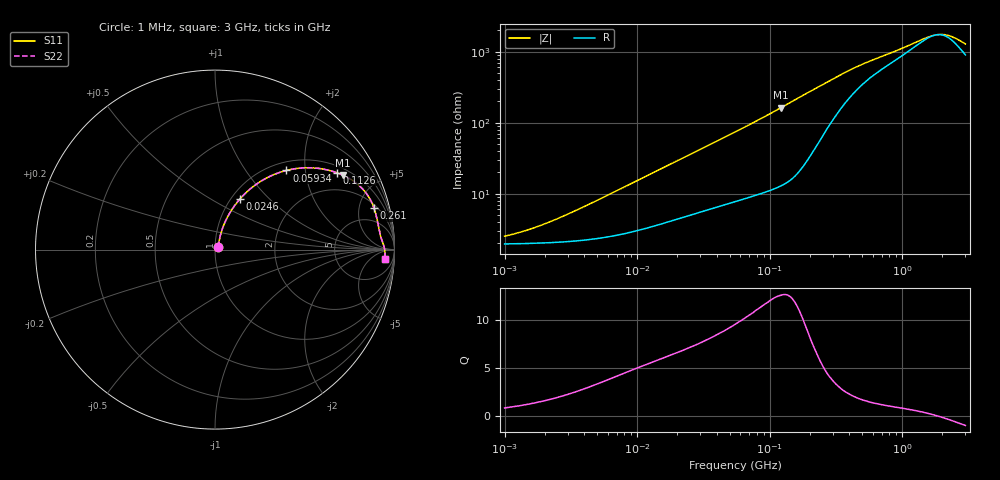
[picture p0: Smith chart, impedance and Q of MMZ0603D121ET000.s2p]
! S-Parameter Data Generated by TDK Corporation
! Copyright(C) 2025 TDK Corporation.
! All Rights Reserved.
! TDK P/N: MMZ0603D121ET000 (Chip Bead)
! Property: |Z|=120ohm at 100MHz
! Size(LxWxT): 0.6x0.3x0.3mm
! Model Type: s2p (Touchstone File Format Version 1.0)
! Frequency: DC=Yes Start=1MHz Stop=3000MHz 202points Log-sweep
! Model Generated on Feb. 6, 2025
! Terms and conditions regarding TDK Simulation Models:
! 1)This simulation model is being provided solely for informational
!  purposes. Please refer to the specifications of the products in
!  terms of detailed characteristics of such products.
! 2)In no event shall TDK Corporation of any of its subsidiaries be
!  liable for any loss or damage arising, directly or indirectly,
!  from any information contained in this simulation model, including,
!  but not limited to loss or damages arising from any inaccuracies,
!  omissions or errors in connection with such information.
! 3)Any and all copyrights on this simulation model are owned by
!  TDK Corporation.  Duplication or redistribution of this simulation
!  model without prior written permission from TDK Corporation
!  is prohibited.
! 4)This simulation model is subject to any modification or change
!  without any prior notice.
! 5)Neither TDK Corporation nor any of its subsidiaries shall make any
!  warranty, express or implied, including but not limited to the
!  correctness, implied warranties of merchantability and fitness for
!  a particular purpose with respect to this simulation models.
! 6)The use of this simulation model shall be deemed to have consented
!  to the terms and conditions hereof.
! Port Assignments:
!  1 ---@@@--- 2
! Applicable Conditions:
!  Temperature = 25 degC
!  DC Bias Current = 0 A
!  Small Signal Operation
# Hz S MA R 50
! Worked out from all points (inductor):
!   201 points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, 1 MHz to 3 GHz, reference 50 ohm
!   read as one part in series: L = 245 nH near 4.398 MHz
!   highest Q = 12.6 at 122 MHz (marker M1), where L = 211 nH
!   self-resonance near 1.818 GHz
!   S11 on the Smith chart (normalised r, x): 1 MHz: 1.04, +0.03; 24.6 MHz: 1.10, +0.69; 59.34 MHz: 1.16, +1.58; 112.6 MHz: 1.24, +2.98; 261 MHz: 2.46, +6.99; 3 GHz: 19, -18
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1000000  0.02469 37.9  0.9806 -0.9  0.9806 -0.9  0.02469 37.9
1377479  0.02886 46.5  0.9803 -1.2  0.9803 -1.2  0.02886 46.5
1897447  0.03537 54.3  0.9798 -1.7  0.9798 -1.7  0.03537 54.3
3900413  0.06306 66.6  0.9767 -3.4  0.9767 -3.4  0.06306 66.6
7703107  0.1161 70.5  0.9675 -6.5  0.9675 -6.5  0.1161 70.5
1.461624e7  0.205 68.6  0.9448 -11.7  0.9448 -11.7  0.205 68.6
2.459509e7  0.317 63.7  0.905 -18.3  0.905 -18.3  0.317 63.7
3.670325e7  0.4317 57.6  0.8511 -25.4  0.8511 -25.4  0.4317 57.6
5.477226e7  0.5661 49.7  0.7673 -34.3  0.7673 -34.3  0.5661 49.7
5.933785e7  0.5942 47.9  0.7464 -36.2  0.7464 -36.2  0.5942 47.9
8.173662e7  0.7045 40.3  0.6494 -44.6  0.6494 -44.6  0.7045 40.3
1.125904e8  0.8021 32.3  0.5362 -53.1  0.5362 -53.1  0.8021 32.3
1.219755e8  0.823 30.3  0.5064 -55.1  0.5064 -55.1  0.823 30.3
1.614254e8  0.8805 23.7  0.4033 -61.3  0.4033 -61.3  0.8805 23.7
2.136344e8  0.9086 18.0  0.3118 -64.2  0.3118 -64.2  0.9086 18.0
2.609752e8  0.9156 14.5  0.2563 -63.7  0.2563 -63.7  0.9156 14.5
4.391493e8  0.9201 7.9  0.1548 -55.0  0.1548 -55.0  0.9201 7.9
8.005644e8  0.9279 4.0  0.09857 -41.0  0.09857 -41.0  0.9279 4.0
1.519029e9  0.9421 0.9  0.06007 -15.0  0.06007 -15.0  0.9421 0.9
1.855641e9  0.9455 -0.1  0.05448 1.9  0.05448 1.9  0.9455 -0.1
2.266846e9  0.9475 -1.2  0.05655 21.3  0.05655 21.3  0.9475 -1.2
3e9  0.9468 -3.0  0.07387 42.5  0.07387 42.5  0.9468 -3.0
